(* Logix 5000 Controller export t; controller t 1768-L45 rev 20.12; software revision 20.01 *)

TASK MainTask (continuous, watchdog 500 ms) : MainProgram

MODULES
   Local : 1768-L45 (1768Ctrl5Slot 0, Compact 0, rev 20.12)
      PLC : 1768-ENBT/A (1768 1, Ethernet 192.168.2.5, rev 2.1)
         gca : ETHERNET-MODULE (Ethernet 192.168.2.16, rev 1.1, Output RPI 10 ms)
END_MODULES

TYPE ControlData_toHFR :
STRUCT
   ModeSelect_Command : SINT;
   ShotNumber_SeqPosition_Request : SINT;
   SequenceNumber_Request : SINT;
   DispenseValveOpen_Request : BOOL;
   RecirculationValveOpen_Request : BOOL;
   SystemStartup_Request : BOOL;
   ParkPump_Request : BOOL;
   HighPressureCirculate_Request_forNVH : BOOL;
   Dispense_Request : BOOL;
   Spare_Bit_Request1 : BOOL;
   Spare_Bit_Request2 : BOOL;
   Bit_Requests_Additional_toHFR : INT;
   FlowPressure_Setpoint_4Dispense : INT;
   FlowSetpoint_4Circulate_p01CCGrmsPerSec : INT;
   ErrorNumberAcknowledgment_CMD : INT;
   Configuratable_CMD1 : INT;
   Configuratable_CMD2 : INT;
   Configuratable_CMD3 : INT;
   Configuratable_CMD4 : INT;
   AmountSetpoint_p01CCGrms_mSecs : DINT;
   TurnON_System_Request : BOOL;
   PLC_Control_Request : BOOL;
   ADM_Lockout_Request : BOOL;
   Red_Tank_ManualFill_Request : BOOL;
   Blue_Tank_ManualFill_Request : BOOL;
   Turn_ON_All_Temp_Zones_Request : BOOL;
   Disable_Dispense_Requests_Command : BOOL;
END_STRUCT
END_TYPE

TYPE DataExchange :
STRUCT
   DataPointer_Last_Serviced_Indication : INT; {access Read Only}
   Data_Input_from_HFR : DINT; {access Read Only}
   DataPointer_Command_toHFR : INT;
   DataOutput_fromPLC : DINT;
END_STRUCT
END_TYPE

TYPE Fluid_Data_fHFR :
STRUCT
   BluePressure_fHFR_p01Bar : INT; {access Read Only}
   RedPressure_fHFR_p01Bar : INT; {access Read Only}
   FlowRate_fHFR_p01CCGrmsPerSec : INT; {access Read Only}
   FlowPressureSetPoint_p01CCGrmsPSecpo1Bar : INT; {access Read Only}
   DispenseDuration_p01Secs : INT; {access Read Only}
   DispensedAmount_p01CCsGrams : DINT; {access Read Only}
   DispenseAmount_SetPoint_po1CCGrms_mSecs : DINT; {access Read Only}
   ModeSelected : SINT; {access Read Only}
   ShotNumberSeqPosition_Current : SINT; {access Read Only}
   Sequence_Selected : SINT; {access Read Only}
   HeartBeat_fromHFR_MCM : BOOL; {access Read Only}
   DispenseValveOpen_DispenseActive_Status : BOOL; {access Read Only}
   RecirculationValveOpen_Indication : BOOL; {access Read Only}
   System_Startup_Active : BOOL; {access Read Only}
   Pumps_Parked_Indication : BOOL; {access Read Only}
   HighPressureCirculation_Active_forNVH : BOOL; {access Read Only}
   ColdStartup_Active : BOOL; {access Read Only}
   Sys_Ready_4Dispense : BOOL; {access Read Only}
   Configurable_Data_InputRegister1 : INT; {access Read Only}
   Configurable_Data_InputRegister2 : INT; {access Read Only}
END_STRUCT
END_TYPE

TYPE Heat_Data_fHFR :
STRUCT
   HeatData_NoLongerUsed1 : BOOL; {access Read Only}
   HeatData_NoLongerUsed2 : BOOL; {access Read Only}
   HeatData_NoLongerUsed3 : BOOL; {access Read Only}
   HeatData_NoLongerUsed4 : BOOL; {access Read Only}
END_STRUCT
END_TYPE

TYPE Inputs_fHFR :
STRUCT
   OldData_ICant_Delete1 : BOOL; {access Read Only}
   OldData_ICant_Delete2 : BOOL; {access Read Only}
   OldData_ICant_Delete3 : BOOL; {access Read Only}
   OldData_ICant_Delete4 : BOOL; {access Read Only}
END_STRUCT
END_TYPE

TYPE Outputs_2HFR :
STRUCT
   OldOutputs_ICantDelete1 : BOOL;
   OldOutputs_ICantDelete2 : BOOL;
   OldOutputs_ICantDelete3 : BOOL;
   OldOutputs_ICantDelete4 : BOOL;
END_STRUCT
END_TYPE

TYPE Status_Bits_fHFR :
STRUCT
   Status_bit0_NotUsed : BOOL; {access Read Only}
   Status_bit1_NotUsed : BOOL; {access Read Only}
   Status_bit2_NotUsed : BOOL; {access Read Only}
   Status_bit3_NotUsed : BOOL; {access Read Only}
END_STRUCT
END_TYPE

VAR_GLOBAL   (* controller tags *)
   ControlData_2HFR : ControlData_toHFR := (ModeSelect_Command := 3, ShotNumber_SeqPosition_Request := 8, SequenceNumber_Request := 26, Bit_Requests_Additional_toHFR := 16#0007, TurnON_System_Request := 1, PLC_Control_Request := 1);
   DataExchange : DataExchange;
   FluidData_fHFR : Fluid_Data_fHFR := (FlowPressureSetPoint_p01CCGrmsPSecpo1Bar := 2500, DispenseAmount_SetPoint_po1CCGrms_mSecs := 8500, ModeSelected := 3, ShotNumberSeqPosition_Current := 8, HeartBeat_fromHFR_MCM := 1, Configurable_Data_InputRegister1 := 25); {access Read Only}
   Heat_Data_fHFR : Heat_Data_fHFR; {access Read Only}
   Inputs_fHFR : Inputs_fHFR; {access Read Only}
   Outputs_2HFR : Outputs_2HFR;
   Status_Bits_fromHFR : Status_Bits_fHFR; {access Read Only}
END_VAR

PROGRAM MainProgram   (* main routine MainRoutine *)
VAR
   sh_3 : BOOL;   // shot #3
END_VAR

ROUTINE MainRoutine   (* ladder *)
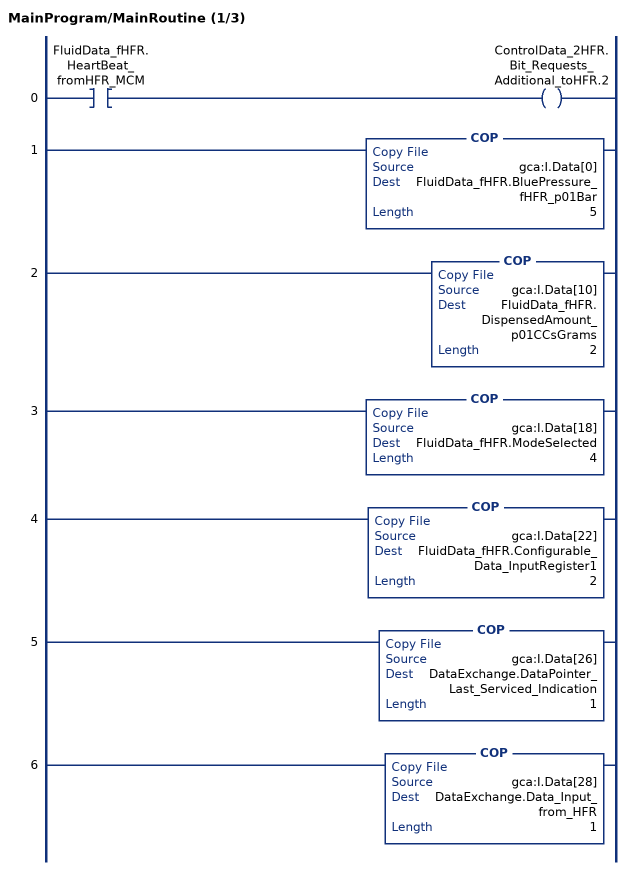
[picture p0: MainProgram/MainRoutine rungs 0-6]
   0: XIC(FluidData_fHFR.HeartBeat_fromHFR_MCM)OTE(ControlData_2HFR.Bit_Requests_Additional_toHFR.2);
   1: COP(gca:I.Data[0],FluidData_fHFR.BluePressure_fHFR_p01Bar,5);
   2: COP(gca:I.Data[10],FluidData_fHFR.DispensedAmount_p01CCsGrams,2);
   3: COP(gca:I.Data[18],FluidData_fHFR.ModeSelected,4);
   4: COP(gca:I.Data[22],FluidData_fHFR.Configurable_Data_InputRegister1,2);
   5: COP(gca:I.Data[26],DataExchange.DataPointer_Last_Serviced_Indication,1);
   6: COP(gca:I.Data[28],DataExchange.Data_Input_from_HFR,1);
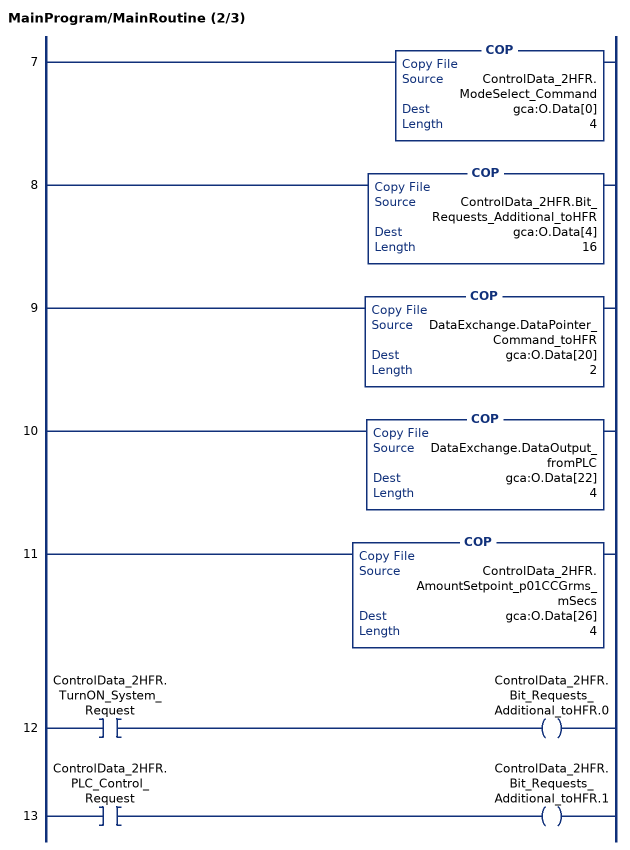
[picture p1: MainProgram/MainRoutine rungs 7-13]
   7: COP(ControlData_2HFR.ModeSelect_Command,gca:O.Data[0],4);
   8: COP(ControlData_2HFR.Bit_Requests_Additional_toHFR,gca:O.Data[4],16);
   9: COP(DataExchange.DataPointer_Command_toHFR,gca:O.Data[20],2);
   10: COP(DataExchange.DataOutput_fromPLC,gca:O.Data[22],4);
   11: COP(ControlData_2HFR.AmountSetpoint_p01CCGrms_mSecs,gca:O.Data[26],4);
   12: XIC(ControlData_2HFR.TurnON_System_Request)OTE(ControlData_2HFR.Bit_Requests_Additional_toHFR.0);
   13: XIC(ControlData_2HFR.PLC_Control_Request)OTE(ControlData_2HFR.Bit_Requests_Additional_toHFR.1);
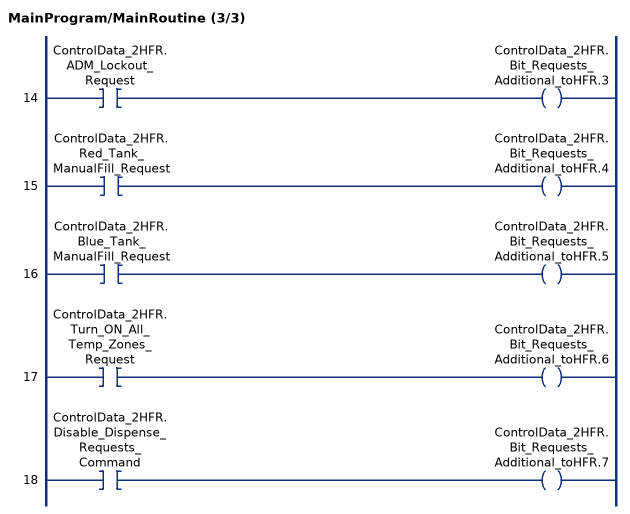
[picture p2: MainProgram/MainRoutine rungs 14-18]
   14: XIC(ControlData_2HFR.ADM_Lockout_Request)OTE(ControlData_2HFR.Bit_Requests_Additional_toHFR.3);
   15: XIC(ControlData_2HFR.Red_Tank_ManualFill_Request)OTE(ControlData_2HFR.Bit_Requests_Additional_toHFR.4);
   16: XIC(ControlData_2HFR.Blue_Tank_ManualFill_Request)OTE(ControlData_2HFR.Bit_Requests_Additional_toHFR.5);
   17: XIC(ControlData_2HFR.Turn_ON_All_Temp_Zones_Request)OTE(ControlData_2HFR.Bit_Requests_Additional_toHFR.6);
   18: XIC(ControlData_2HFR.Disable_Dispense_Requests_Command)OTE(ControlData_2HFR.Bit_Requests_Additional_toHFR.7);
END_ROUTINE
END_PROGRAM
